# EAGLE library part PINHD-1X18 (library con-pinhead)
PIN HEADER
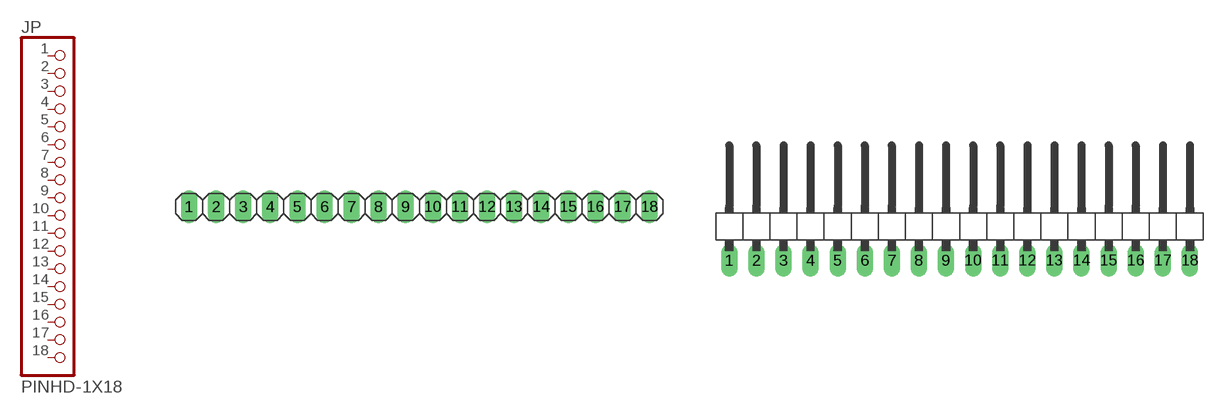
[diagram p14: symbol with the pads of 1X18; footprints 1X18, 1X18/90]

Designator prefix JP

## PINHD-1X18_2.54  [1X18]
1  1  pas
2  2  pas
3  3  pas
4  4  pas
5  5  pas
6  6  pas
7  7  pas
8  8  pas
9  9  pas
10  10  pas
11  11  pas
12  12  pas
13  13  pas
14  14  pas
15  15  pas
16  16  pas
17  17  pas
18  18  pas

## PINHD-1X18_2.54-90°  [1X18/90]
Pads as for 1X18

## PINHD-1X18_2.00  [1X18M]
Pads as for 1X18

## PINHD-1X18_2.54-SMD  [1X18SMD]
Pads as for 1X18

## PINHD-1X18_2.54-SMD-90°  [1X18SMD/90]
Pads as for 1X18

## Footprint 1X18 (pad centres in mm)
PIN HEADER - 2.54
drill 1.016 long: 1 -21.59,0; 2 -19.05,0; 3 -16.51,0; 4 -13.97,0; 5 -11.43,0; 6 -8.89,0; 7 -6.35,0; 8 -3.81,0; 9 -1.27,0; 10 1.27,0; 11 3.81,0; 12 6.35,0; 13 8.89,0; 14 11.43,0; 15 13.97,0; 16 16.51,0; 17 19.05,0; 18 21.59,0

## Footprint 1X18/90 (pad centres in mm)
PIN HEADER - 2.54 90°
drill 1.016 long: 1 -21.59,-3.81; 2 -19.05,-3.81; 3 -16.51,-3.81; 4 -13.97,-3.81; 5 -11.43,-3.81; 6 -8.89,-3.81; 7 -6.35,-3.81; 8 -3.81,-3.81; 9 -1.27,-3.81; 10 1.27,-3.81; 11 3.81,-3.81; 12 6.35,-3.81; 13 8.89,-3.81; 14 11.43,-3.81; 15 13.97,-3.81; 16 16.51,-3.81; 17 19.05,-3.81; 18 21.59,-3.81

## Footprint 1X18M (pad centres in mm)
PIN HEADER - 2
drill 0.914 square: 1 -17,0
drill 0.914: 2 -15,0; 3 -13,0; 4 -11,0; 5 -9,0; 6 -7,0; 7 -5,0; 8 -3,0; 9 -1,0; 10 1,0; 11 3,0; 12 5,0; 13 7,0; 14 9,0; 15 11,0; 16 13,0; 17 15,0; 18 17,0

## Footprint 1X18SMD (pad centres in mm)
PIN HEADER - 2.54 SMD
smd 1.016 x 3.302: 1 -1.27,1.27; 2 1.27,-1.27; 3 3.81,1.27; 4 6.35,-1.27; 5 8.89,1.27; 6 11.43,-1.27; 7 13.97,1.27; 8 16.51,-1.27; 9 19.05,1.27; 10 21.59,-1.27; 11 24.13,1.27; 12 26.67,-1.27; 13 29.21,1.27; 14 31.75,-1.27; 15 34.29,1.27; 16 36.83,-1.27; 17 39.37,1.27; 18 41.91,-1.27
